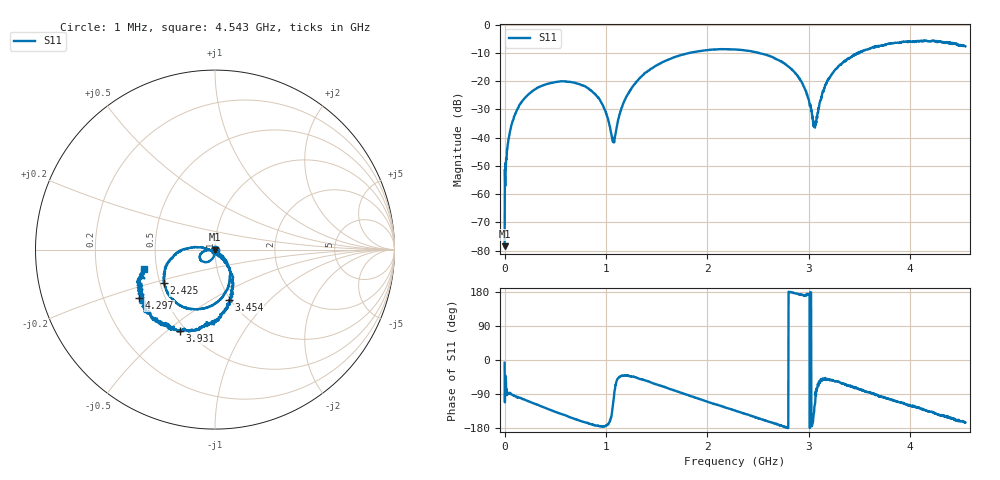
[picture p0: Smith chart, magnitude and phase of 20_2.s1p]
# HZ S RI R 50
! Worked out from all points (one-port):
!   1515 points, 1 MHz to 4.543 GHz, reference 50 ohm
!   lowest |S11| = -78.4 dB at 1 MHz (marker M1), VSWR 1.00, Z = 50 - j0.00149 ohm
!   |S11| at or under -10 dB: start of sweep to 1.826 GHz; 2.497517 GHz to 2.502425 GHz (4.908 MHz wide, 0.196 % of centre); 2.506 GHz to 3.483 GHz (977.2 MHz wide, 32.6 % of centre)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
!   S11 on the Smith chart (normalised r, x): 1 MHz: 1.00, -0.00; 2.425 GHz: 0.52, -0.22; 3.454 GHz: 0.98, -0.61; 3.931 GHz: 0.47, -0.56; 4.297 GHz: 0.36, -0.26; 4.543 GHz: 0.42, -0.11
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1000000  0.000119 -1.49e-05
2.5e7  -0.000307 -0.0062
3.1e7  0.000514 -0.00741
6.1e7  0.00044 -0.0144
1.15e8  -0.00367 -0.0284
3.01e8  -0.0311 -0.0642
5.71e8  -0.0796 -0.0592
7.9e8  -0.0784 -0.0219
9.13e8  -0.0533 -0.0063
9.94e8  -0.0293 -0.00283
1.072e9  -0.00314 -0.00812
1.138e9  0.0192 -0.0182
1.219e9  0.0446 -0.0395
1.345e9  0.0757 -0.092
1.705e9  0.0347 -0.2746
2.272e9  -0.249 -0.2633
2.425e9  -0.285 -0.1856
2.641e9  -0.2554 -0.0673
2.842e9  -0.1534 0.00472
2.956e9  -0.0748 0.0145
3.061e9  -0.00638 -0.0135
3.181e9  0.0648 -0.0767
3.409e9  0.0974 -0.2414
3.454e9  0.0767 -0.2827
3.931e9  -0.1933 -0.4528
3.976e9  -0.229 -0.4298
4.297e9  -0.4225 -0.27
4.543e9  -0.3982 -0.1071
